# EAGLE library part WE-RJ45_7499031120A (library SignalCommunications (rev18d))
Order Code 7499031120A Design THT xBase-T 10/100 Base-T Ports 1x4 HORIZONTAL Application Standard Tab Position DOWN LED (Left-Right) YELLOW-GREEN EMI Fingers Yes Details see: http://katalog.we-online.de/en/pbs/WE-LAN_RJ45/7499031120A? Updated by Yingchun Shan 2016-08-29 2016(C) Würth Elektronik
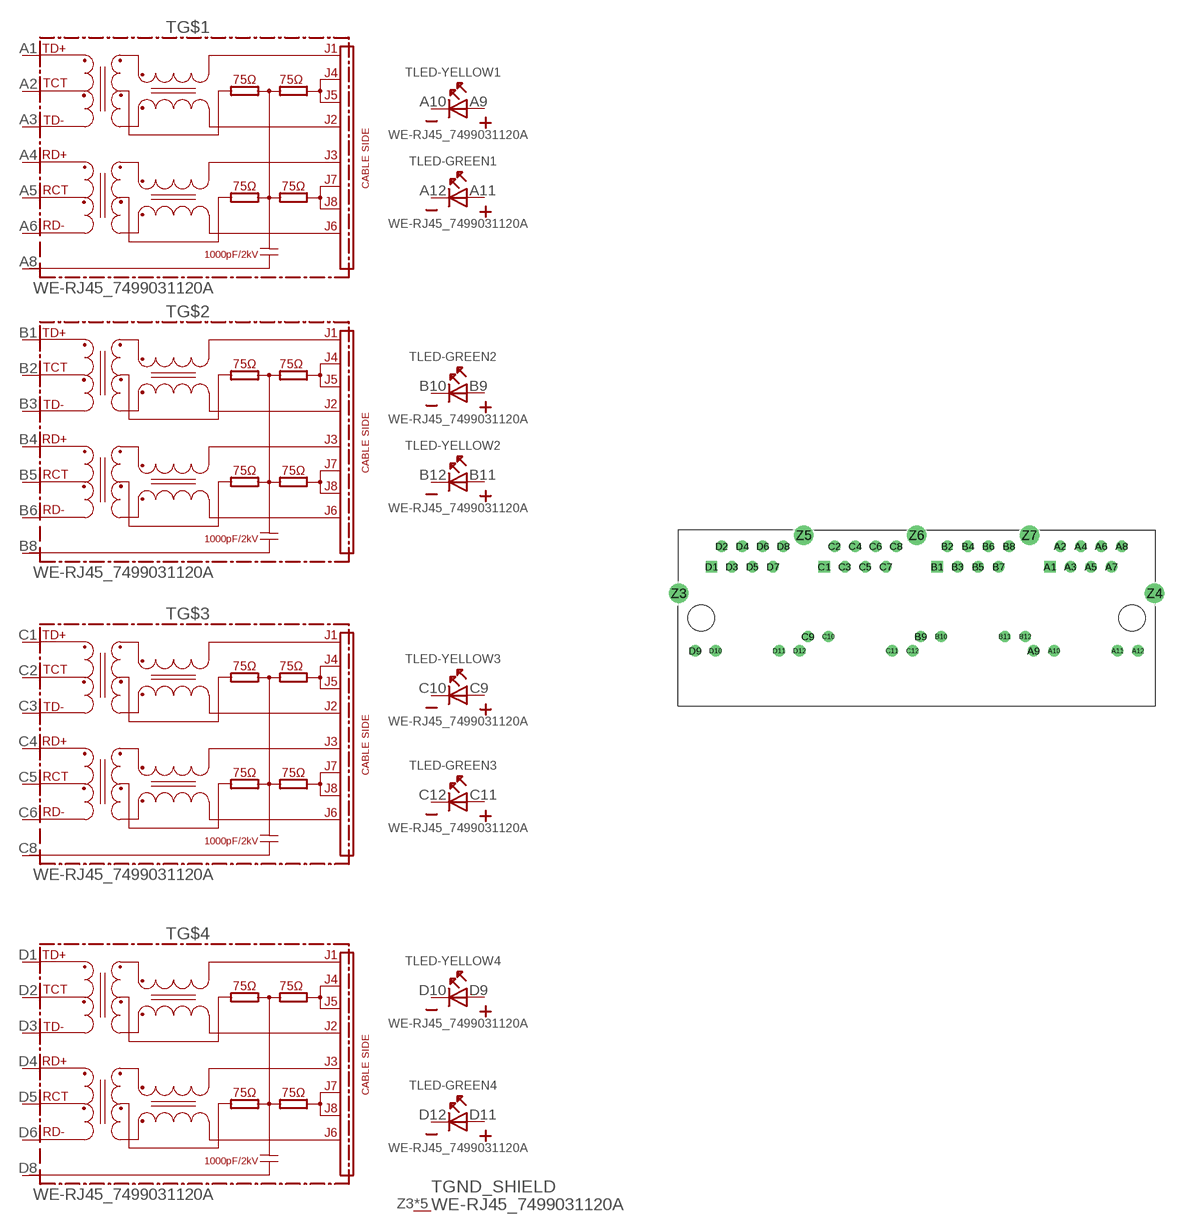
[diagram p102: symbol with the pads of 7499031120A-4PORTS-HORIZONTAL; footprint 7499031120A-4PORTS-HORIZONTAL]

Designator prefix T; gates LED-YELLOW2=LED2PIN LED-GREEN1=LED2PIN LED-GREEN2=LED2PIN LED-YELLOW1=LED2PIN LED-YELLOW3=LED2PIN LED-GREEN3=LED2PIN LED-YELLOW4=LED2PIN LED-GREEN4=LED2PIN GND_SHIELD=GND_PIN G$1=74990X-THT-10/100-T G$2=74990X-THT-10/100-T G$3=74990X-THT-10/100-T G$4=74990X-THT-10/100-T

## WE-RJ45_7499031120A (COMPANY-URL: http://www.we-online.de; CREATED-BY: Christin Zierenner; CREATED-DATE: AUG 2012; DATASHEET-URL: http://katalog.we-online.de/kataloge/eisos/media/pdf/7499031120A.pdf; MANUFACTURER: Würth Elektronik eiSos GmbH)  [7499031120A-4PORTS-HORIZONTAL]
A1  G$1:TD+
A2  G$1:TCT
A3  G$1:TD-
A4  G$1:RD+
A5  G$1:RCT
A6  G$1:RD-
A8  G$1:8
A9  LED-YELLOW1:A  pas
A10  LED-YELLOW1:K  pas
A11  LED-GREEN1:A  pas
A12  LED-GREEN1:K  pas
B1  G$2:TD+
B2  G$2:TCT
B3  G$2:TD-
B4  G$2:RD+
B5  G$2:RCT
B6  G$2:RD-
B8  G$2:8
B9  LED-GREEN2:A  pas
B10  LED-GREEN2:K  pas
B11  LED-YELLOW2:A  pas
B12  LED-YELLOW2:K  pas
C1  G$3:TD+
C2  G$3:TCT
C3  G$3:TD-
C4  G$3:RD+
C5  G$3:RCT
C6  G$3:RD-
C8  G$3:8
C9  LED-YELLOW3:A  pas
C10  LED-YELLOW3:K  pas
C11  LED-GREEN3:A  pas
C12  LED-GREEN3:K  pas
D1  G$4:TD+
D2  G$4:TCT
D3  G$4:TD-
D4  G$4:RD+
D5  G$4:RCT
D6  G$4:RD-
D8  G$4:8
D9  LED-YELLOW4:A  pas
D10  LED-YELLOW4:K  pas
D11  LED-GREEN4:A  pas
D12  LED-GREEN4:K  pas
Z3  GND_SHIELD:1  pwr
Z4  GND_SHIELD:1  pwr
Z5  GND_SHIELD:1  pwr
Z6  GND_SHIELD:1  pwr
Z7  GND_SHIELD:1  pwr

## Footprint 7499031120A-4PORTS-HORIZONTAL (pad centres in mm)
MAX HEIGHT=13.50mm PORTS----1X4 HORIZONTAL LED --YES
drill 0.89 square: A1 16.51,6.35; B1 2.54,6.35; C1 -11.43,6.35; D1 -25.4,6.35
drill 0.89: A2 17.78,8.89; A3 19.05,6.35; A4 20.32,8.89; A5 21.59,6.35; A6 22.86,8.89; A7 24.13,6.35; A8 25.4,8.89; A9 14.48,-4.06; A10 17.02,-4.06; A11 24.88,-4.06; A12 27.42,-4.06; B2 3.81,8.89; B3 5.08,6.35; B4 6.35,8.89; B5 7.62,6.35; B6 8.89,8.89; B7 10.16,6.35; B8 11.43,8.89; B9 0.51,-2.29; B10 3.05,-2.29; B11 10.92,-2.29; B12 13.46,-2.29; C2 -10.16,8.89; C3 -8.89,6.35; C4 -7.62,8.89; C5 -6.35,6.35; C6 -5.08,8.89; C7 -3.81,6.35; C8 -2.54,8.89; C9 -13.46,-2.29; C10 -10.92,-2.29; C11 -3.05,-4.06; C12 -0.51,-4.06; D2 -24.13,8.89; D3 -22.86,6.35; D4 -21.59,8.89; D5 -20.32,6.35; D6 -19.05,8.89; D7 -17.78,6.35; D8 -16.51,8.89; D9 -27.42,-4.06; D10 -24.88,-4.06; D11 -17.02,-4.06; D12 -14.48,-4.06
drill 1.63: Z3 -29.455,3.05; Z4 29.455,3.05; Z5 -13.97,10.24; Z6 0,10.24; Z7 13.97,10.24
hole 3.25 at -26.67,0
hole 3.25 at 26.67,0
